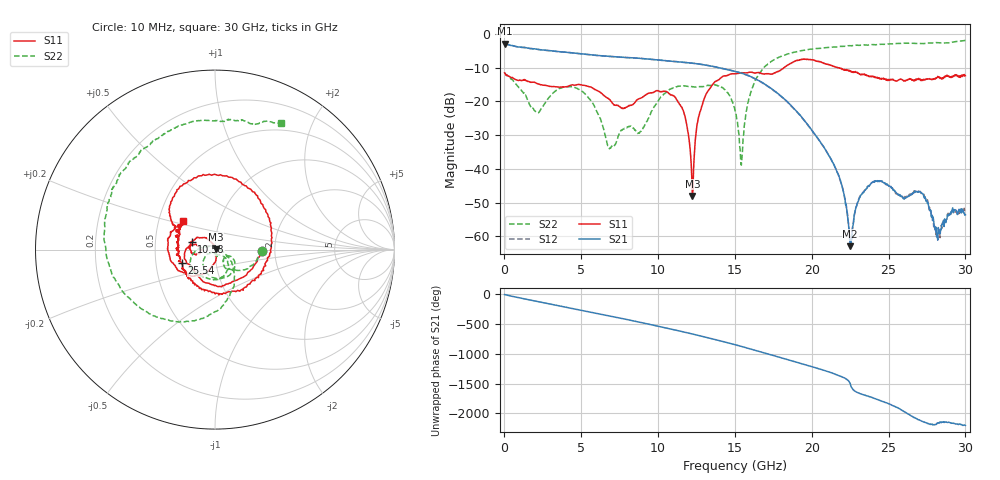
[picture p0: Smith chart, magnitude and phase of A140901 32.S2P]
!  2-Port S-parameters saved by WinCal
! VAR MeasName=S-Parameters (CALIBRATED_DATA) read from VNA (N5244A)
! VAR MeasDate=11/3/2014 9:29:24 AM
! VAR NAME=A140901 32
! VAR FILENAME=A140901 32.S2P
! VAR DATE=11/3/2014 9:29:24 AM
! VAR PHYS_PORTS=1,2
# Hz S RI R 50
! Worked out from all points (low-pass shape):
!   801 points, 10 MHz to 30 GHz, reference 50 ohm
!   highest |S21| = -2.91 dB at 10 MHz (marker M1); lowest = -62.9 dB at 22.5 GHz (marker M2)
!   |S21| within 3 dB of the highest: start of sweep to 4.916 GHz
!   lowest |S11| = -48.0 dB at 12.23 GHz (marker M3), VSWR 1.01, Z = 50.3 + j0.203 ohm
!   |S11| at or under -10 dB: start of sweep to 18.22 GHz; 21.66 GHz to end of sweep
!   |S22| runs from -38.9 to -2.0 dB; largest |S21 - S12| = 0.0033
!   S11 on the Smith chart (normalised r, x): 10 MHz: 1.72, -0.03; 10.58 GHz: 0.77, +0.07; 25.54 GHz: 0.68, -0.11; 30 GHz: 0.67, +0.23
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1e7  0.2634 -0.00768  0.7152 -0.012  0.714 -0.0117  0.2637 -0.00598
1.434525e9  0.00242 -0.1995  0.0968 -0.6103  0.0967 -0.6097  0.0549 -0.0999
2.971512e9  -0.1168 -0.1186  -0.5296 -0.186  -0.5292 -0.1863  0.1046 -0.056
5.033325e9  -0.1702 -0.0371  -0.0209 0.5023  -0.0205 0.5019  -0.0431 -0.1345
6.870212e9  -0.1021 0.0248  0.4602 -0.0234  0.4603 -0.0231  -0.0103 -0.0175
8.444688e9  -0.0906 -0.0214  0.0223 -0.4373  0.0232 -0.4367  0.0116 -0.0369
1.001916e10  -0.1425 0.00986  -0.4073 -0.0365  -0.4068 -0.0356  0.0705 -0.0732
1.058148e10  -0.1299 0.0438  -0.3549 0.1797  -0.3545 0.1803  0.0648 -0.1237
1.166861e10  -0.0396 0.0572  0.00307 0.3766  0.00225 0.3771  -0.0161 -0.1684
1.223092e10  0.00341 0.00202  0.2069 0.3012  0.2073 0.3011  -0.0461 -0.158
1.309314e10  -0.0361 -0.1175  0.3441 0.00845  0.3437 0.00822  -0.085 -0.1458
1.5005e10  -0.2526 -0.0382  -0.1557 -0.2287  -0.157 -0.2271  -0.0718 0.0114
1.541736e10  -0.2632 0.00173  -0.2328 -0.117  -0.2345 -0.1158  0.00636 0.00935
1.669194e10  -0.239 0.1012  -0.0768 0.1787  -0.0742 0.1784  0.0737 -0.2635
2.002832e10  0.0954 0.4018  -0.0266 -0.0253  -0.026 -0.0257  -0.5819 -0.1085
2.175275e10  0.3133 0.00872  0.00186 0.00773  0.00172 0.00773  -0.6027 0.2317
2.25025e10  0.2213 -0.166  0.00041 -0.000585  0.000339 -0.000682  -0.5644 0.3491
2.347718e10  0.0192 -0.2445  -0.00115 0.00468  -0.00127 0.00465  -0.4678 0.4996
2.501416e10  -0.1648 -0.1179  0.00432 -0.0034  0.00451 -0.00351  -0.2747 0.6522
2.553899e10  -0.1841 -0.0743  -0.000676 -0.00421  -0.000777 -0.00424  -0.2043 0.6895
2.82006e10  -0.2201 0.0771  0.000876 2.69e-05  0.00111 -3.33e-05  0.1559 0.7209
3e10  -0.1762 0.1613  0.00152 -0.00142  0.00156 -0.00155  0.3678 0.7032
